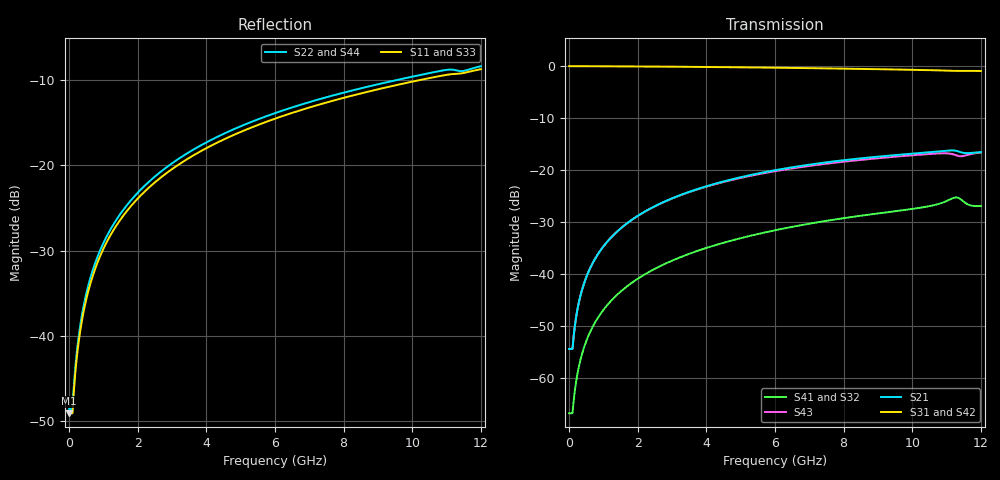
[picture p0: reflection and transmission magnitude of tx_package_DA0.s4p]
! Created Mon Sep 08 15:26:53 2014
# hz S db R 50
! 4 Port Network Data from SP1.SP block
! freq  dbS11  angS11  dbS12  angS12  dbS13  angS13  dbS14  angS14
!  dbS21  angS21  dbS22  angS22  dbS23  angS23  dbS24  angS24
!  dbS31  angS31  dbS32  angS32  dbS33  angS33  dbS34  angS34
!  dbS41  angS41  dbS42  angS42  dbS43  angS43  dbS44  angS44
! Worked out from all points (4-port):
!   1201 points, 1 MHz to 12 GHz, reference 50 ohm
!   strongest paths, dB at 1 MHz, 3.001 GHz, 6.001 GHz, 9.001 GHz, 12 GHz:
!     S31: 0.0, -0.1, -0.3, -0.6, -0.9
!     S42: 0.0, -0.1, -0.3, -0.6, -1.0
!     S21: -54.4, -25.4, -20.0, -17.4, -16.5
!     S43: -54.4, -25.5, -20.2, -17.7, -16.6
!     S41: -66.7, -37.4, -31.6, -28.3, -26.9
!     S32: -66.6, -37.4, -31.6, -28.4, -27.1
!   lowest |S11| = -49.1 dB at 1 MHz (marker M1), VSWR 1.01, Z = 50.1 + j0.328 ohm
!   |S11| at or under -10 dB: start of sweep to 10.18 GHz
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1000000  -49.13 69.3  -54.36 85.9  -0.01 -0.6  -66.74 -100.5
         -54.36 85.9  -48.62 72.0  -66.64 -100.6  -0.01 -0.6
         -0.01 -0.6  -66.64 -100.6  -49.12 69.0  -54.37 86.1
         -66.74 -100.5  -0.01 -0.6  -54.37 86.1  -48.64 71.6
3.91e8  -37.86 83.1  -42.71 85.7  -0.02 -2.3  -55.03 -97.3
        -42.71 85.7  -37.21 83.9  -55.02 -97.2  -0.02 -2.3
        -0.02 -2.3  -55.02 -97.2  -37.85 80.7  -42.70 86.2
        -55.03 -97.3  -0.02 -2.3  -42.70 86.2  -37.19 81.6
8.11e8  -31.59 84.3  -36.46 83.2  -0.03 -4.7  -48.68 -101.6
        -36.46 83.2  -30.92 84.7  -48.68 -101.6  -0.03 -4.7
        -0.03 -4.7  -48.68 -101.6  -31.59 79.4  -36.45 84.1
        -48.68 -101.6  -0.03 -4.7  -36.45 84.1  -30.92 79.9
2.631e9  -21.56 80.9  -26.50 71.4  -0.09 -15.1  -38.53 -124.7
         -26.50 71.4  -20.87 80.8  -38.54 -124.2  -0.10 -15.1
         -0.09 -15.1  -38.54 -124.2  -21.59 65.1  -26.53 74.1
         -38.53 -124.7  -0.10 -15.1  -26.53 74.1  -20.91 65.7
6.511e9  -13.81 70.9  -19.44 46.2  -0.35 -36.8  -30.89 -174.0
         -19.44 46.2  -13.17 70.2  -30.93 -172.8  -0.37 -36.9
         -0.35 -36.8  -30.93 -172.8  -13.90 33.0  -19.65 54.1
         -30.89 -174.0  -0.37 -36.9  -19.65 54.1  -13.26 33.9
1.1251e10  -9.25 57.0  -16.25 12.4  -0.92 -62.5  -25.25 123.4
           -16.25 12.4  -8.80 54.1  -25.18 124.4  -1.11 -62.5
           -0.92 -62.5  -25.18 124.4  -9.40 -6.0  -17.08 31.2
           -25.25 123.4  -1.11 -62.5  -17.08 31.2  -8.83 -6.6
1.2e10  -8.69 56.0  -16.54 10.9  -0.95 -66.5  -26.90 113.0
        -16.54 10.9  -8.34 55.3  -27.13 114.3  -1.02 -66.0
        -0.95 -66.5  -27.13 114.3  -8.95 -10.3  -16.59 33.9
        -26.90 113.0  -1.02 -66.0  -16.59 33.9  -8.58 -9.4
